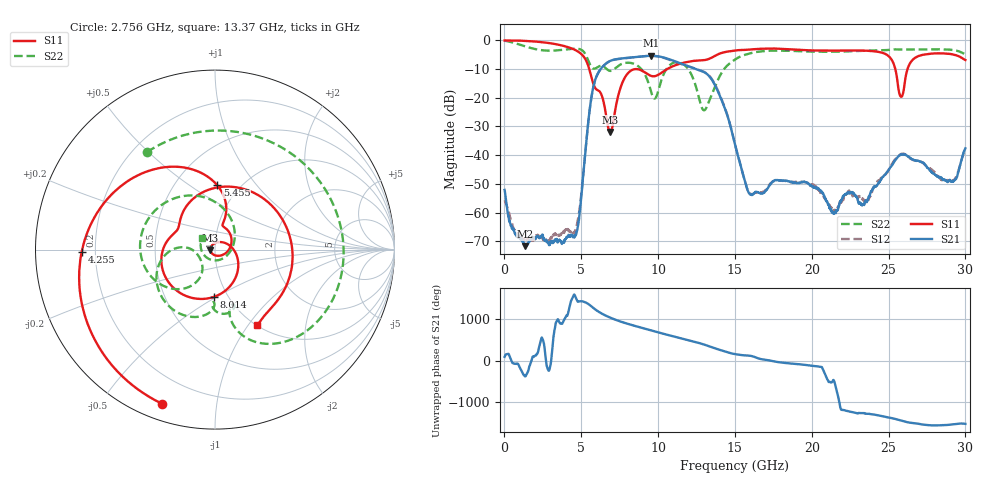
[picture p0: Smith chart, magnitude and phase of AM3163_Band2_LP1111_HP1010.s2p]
!Agilent Technologies,E8364B,MY43040894,A.07.50.67
!Agilent E8364B: A.07.50.67
!Date: Thursday, August 20, 2020 12:09:43
!Correction: S11(Full 2 Port(1,2))
!S21(Full 2 Port(1,2))
!S12(Full 2 Port(1,2))
!S22(Full 2 Port(1,2))
!S2P File: Measurements: S11, S21, S12, S22:
# Hz S  dB  R 50
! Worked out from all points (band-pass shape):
!   3201 points, 10 MHz to 30 GHz, reference 50 ohm
!   highest |S21| = -5.39 dB at 9.541 GHz (marker M1); lowest = -71.7 dB at 1.35 GHz (marker M2)
!   |S21| within 3 dB of the highest: 6.537 GHz to 11.64 GHz (5.107 GHz wide, 56.2 % of centre)
!   lowest |S11| = -31.9 dB at 6.889 GHz (marker M3), VSWR 1.05, Z = 47.5 - j0.158 ohm
!   |S11| at or under -10 dB: 5.518 GHz to 10.59 GHz (5.073 GHz wide, 63 % of centre); 25.44 GHz to 26.23 GHz (795.4 MHz wide, 3.08 % of centre)
!   |S22| runs from -24.4 to -0.1 dB; largest |S21 - S12| = 0.012
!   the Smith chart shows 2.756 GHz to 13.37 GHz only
!   S11 on the Smith chart (normalised r, x): 2.756 GHz: 0.07, -0.71; 4.255 GHz: 0.15, -0.01; 5.455 GHz: 0.79, +0.65; 8.014 GHz: 0.86, -0.49; 13.37 GHz: 1.01, -1.11
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1e7  -0.05 -2.5  -52.09 92.7  -55.70 -11.8  -0.14 -6.7
1.350178e9  -0.17 -52.5  -71.68 -19.2  -69.27 16.8  -2.10 -124.1
2.755959e9  -0.84 -109.1  -69.99 -127.8  -69.95 166.1  -3.58 124.9
4.255459e9  -2.59 -179.2  -68.33 -108.8  -66.73 -77.2  -3.01 17.1
5.014581e9  -4.83 130.1  -53.66 -1.3  -52.73 -0.7  -3.34 -42.2
5.455059e9  -8.91 88.0  -28.44 -66.5  -28.52 -66.9  -7.05 -75.8
6.888956e9  -31.94 -176.2  -7.15 -38.5  -7.18 -38.6  -10.65 -91.9
8.013581e9  -11.59 -91.2  -6.10 173.9  -6.15 174.2  -7.79 -122.5
9.541197e9  -12.38 155.9  -5.39 14.2  -5.38 14.1  -17.85 -180.0
1.000979e10  -12.01 141.4  -5.58 -33.8  -5.60 -34.2  -17.60 -122.1
1.136871e10  -8.23 51.1  -7.84 -166.2  -8.04 -165.0  -7.64 162.2
1.337429e10  -6.32 -60.8  -12.79 -17.1  -12.62 -15.4  -20.42 138.5
1.5005e10  -3.55 -132.0  -36.37 160.7  -36.22 160.2  -6.69 -112.2
1.598905e10  -3.20 -173.2  -53.65 120.0  -53.38 118.8  -4.53 -171.6
1.787279e10  -2.90 98.3  -48.78 -36.5  -48.90 -37.8  -3.57 92.1
2.000958e10  -3.51 -9.9  -50.78 -121.8  -50.25 -123.1  -3.93 -9.4
2.231506e10  -3.54 -100.0  -53.31 -136.5  -53.08 -113.1  -3.86 -93.8
2.500479e10  -5.51 157.8  -45.21 65.6  -45.05 67.7  -3.35 -167.6
2.582014e10  -19.66 171.9  -39.87 -9.6  -39.56 -6.5  -3.20 170.3
2.727278e10  -4.99 157.2  -42.65 -106.8  -42.88 -105.1  -3.18 133.0
2.919402e10  -4.92 84.3  -49.13 -98.1  -48.94 -102.8  -3.37 78.7
3e10  -6.86 54.2  -37.61 -87.9  -37.88 -87.4  -4.84 55.3
